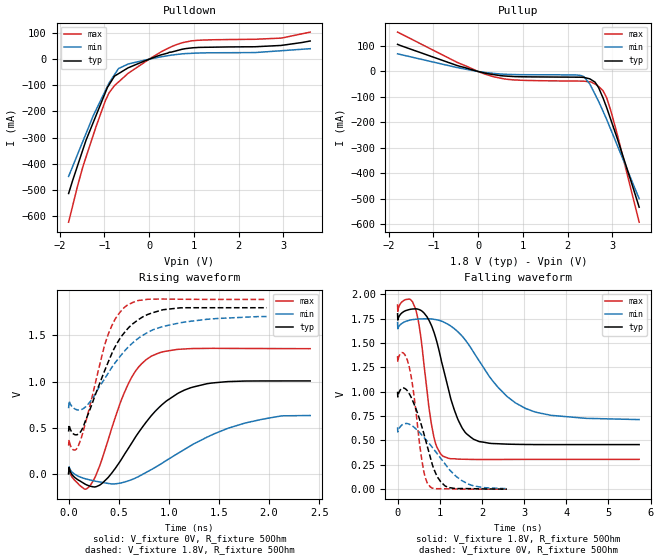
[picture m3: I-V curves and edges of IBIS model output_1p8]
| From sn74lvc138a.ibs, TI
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|   output_1p8 Model
[Model]   output_1p8
Model_type   Output
Polarity   Non-Inverting
Vmeas = 0.9
Vref = 0.9
Cref = 2pF
Rref = 50
|   typ   min   max
|   (nom PVT)   (fast PVT)   (slow PVT)
|C_comp from frequency sweep method (F=5MHz)
|C_comp   6.350e-12   6.256e-12   7.540e-12
|ON state : BUFFER OUTPUT TURNED HIGH
|C_comp   6.350e-12   6.256e-12   7.540e-12
|OFF state: BUFFER OUTPUT TURNED LOW
|C_comp   9.360e-12   9.345e-12   9.377e-12
|C_comp from LC tank measurement(L=1nH)
|Resonant Frequency(Hz)   2.130e+09   2.150e+09   2.080e+09
C_comp   5.589e-12   5.485e-12   5.861e-12
|ON state : BUFFER OUTPUT TURNED HIGH
|Resonant Frequency(Hz)   2.130e+09   2.150e+09   2.080e+09
|C_comp   5.589e-12   5.485e-12   5.861e-12
|OFF state: BUFFER OUTPUT TURNED LOW
|Resonant Frequency(Hz)   2.190e+09   2.210e+09   2.120e+09
|C_comp   5.287e-12   5.191e-12   5.642e-12
| Where nom  PVT is Nominal Process, 1.8V, 27C
|   Fast PVT is Strong Process,  1.89V, -40C
|   Slow PVT is Weak Process,   1.71V, 125C
[Voltage Range]   1.8   1.71   1.89
|Ambient Temperature   25   85   -40
|Junction Temperature
[Temperature Range]   27   125   -40
[Pullup Reference]   1.8   1.71   1.89
[Pulldown Reference]   0   0   0
[Power Clamp Reference]   1.8   1.71   1.89
[GND Clamp Reference]   0   0   0
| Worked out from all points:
|   slope of the pulldown table from 0 to 0.27 V, typ, clamps not added: 16.1 ohm
|   slope of the pullup table from 0 to 0.27 V, typ, clamps not added: 26.3 ohm
|   falling waveform, V_fixture 1.8V, R_fixture 50Ohm: 20-80 % time 503ps typ, 1.07ns min, 274ps max; typ from 1.8 V to 0.457 V
|   rising waveform, V_fixture 0V, R_fixture 50Ohm: 20-80 % time 446ps typ, 676ps min, 284ps max; typ from 0 V to 1.01 V
|   rising waveform, V_fixture 1.8V, R_fixture 50Ohm: 20-80 % time 335ps typ, 458ps min, 233ps max; typ from 0.457 V to 1.8 V
|   falling waveform, V_fixture 0V, R_fixture 50Ohm: 20-80 % time 412ps typ, 719ps min, 240ps max; typ from 1 V to 0 V
[Pulldown]
|   Voltage   I(typ)   I(min)   I(max)
-1.8V     -514.4mA   -448.9mA   -624.4mA
-1.482V   -347mA     -314.7mA   -412.2mA
-1.248V   -241.8mA   -216.2mA   -290.4mA
-980.9mV  -128.6mA   -121.3mA   -160mA
-897.8mV  -98.72mA   -91.84mA   -129.5mA
-774mV    -64.74mA   -59.18mA   -101.1mA
-685.7mV  -55.53mA   -36.01mA   -87.51mA
-470.6mV  -33.13mA   -18.62mA   -54.29mA
258.9mV   16.22mA    8.746mA    27.32mA
761.7mV   38.89mA    20.81mA    63.97mA
2.948V    52.67mA    32.41mA    80.78mA
3.6V      69.74mA    40.27mA    103.9mA
[Pullup]
|   Voltage   I(typ)   I(min)   I(max)
-1.8V     106.4mA    69.22mA    154.5mA
-470.6mV  23.41mA    15.43mA    35.98mA
332.6mV   -11.89mA   -7.173mA   -19.91mA
786.2mV   -19.78mA   -12.05mA   -32.97mA
2.291V    -22.48mA   -15.36mA   -37.74mA
2.367V    -23.31mA   -20.71mA   -37.9mA
2.497V    -28.83mA   -48.86mA   -40.43mA
2.663V    -55.08mA   -106.6mA   -54.04mA
2.79V     -102.6mA   -154.8mA   -74.48mA
2.871V    -140.4mA   -186.9mA   -102.1mA
2.967V    -189.6mA   -228.1mA   -154.2mA
3.6V      -532.3mA   -499.1mA   -591.2mA
[Ramp]
R_load = 50
|   typ   min   max
dV/dt_r   0.602271/4.41058e-10   0.391369/7.13501e-10   0.813764/2.83941e-10
dV/dt_f   0.805639/5.02765e-10   0.599447/1.06929e-09   0.950749/2.73761e-10
[Falling Waveform]
V_fixture = 1.8V
V_fixture_min = 1.71V
V_fixture_max = 1.89V
R_fixture = 50Ohm
|   Time   V(typ)   V(min)   V(max)
0s        1.8V       1.71V      1.89V
425ps     1.851V     1.744V     1.851V
540ps     1.838V     1.747V     1.599V
815ps     1.668V     1.746V     639.1mV
1.08ns    1.246V     1.718V     337.6mV
1.44ns    706.8mV    1.611V     307.9mV
1.935ns   488.3mV    1.316V     304.4mV
2.59ns    462mV      953.9mV    304.9mV
3.225ns   457.7mV    797.7mV    305.4mV
5.73ns    457.3mV    714.1mV    305.4mV
[Rising Waveform]
V_fixture = 0V
V_fixture_min = 0V
V_fixture_max = 0V
R_fixture = 50Ohm
|   Time   V(typ)   V(min)   V(max)
0s        108.6pV    12.82nV    54.42pV
5ps       69.56mV    74.84mV    62.58mV
115ps     -79.37mV   -35.53mV   -129.9mV
215ps     -134.8mV   -68.02mV   -127.7mV
390ps     -45.68mV   -104.4mV   351mV
590ps     265.1mV    -78.88mV   962.1mV
825ps     629.8mV    44.73mV    1.274V
1.09ns    871.4mV    220.5mV    1.349V
1.38ns    976.1mV    396.3mV    1.359V
2.41ns    1.006V     631.4mV    1.356V
[Rising Waveform]
V_fixture = 1.8V
V_fixture_min = 1.71V
V_fixture_max = 1.89V
R_fixture = 50Ohm
|   Time   V(typ)   V(min)   V(max)
0s        457.3mV    710.9mV    305.4mV
5ps       529.6mV    790.3mV    369.8mV
45ps      434.6mV    716.2mV    260.8mV
100ps     432.4mV    690.9mV    310.8mV
210ps     688.1mV    773.6mV    725.7mV
380ps     1.172V     1.065V     1.465V
465ps     1.379V     1.204V     1.677V
570ps     1.548V     1.345V     1.816V
945ps     1.779V     1.598V     1.894V
1.975ns   1.8V       1.704V     1.89V
[Falling Waveform]
V_fixture = 0V
V_fixture_min = 0V
V_fixture_max = 0V
R_fixture = 50Ohm
|   Time   V(typ)   V(min)   V(max)
0s        1V         634mV      1.366V
140ps     1.038V     668.7mV    1.397V
265ps     987.7mV    668.6mV    1.274V
370ps     895.4mV    642.6mV    1.022V
615ps     582.4mV    536.3mV    198.2mV
775ps     329.4mV    454.6mV    22.86mV
955ps     118.6mV    355.2mV    4.503mV
1.215ns   15.76mV    208mV      2.754mV
1.77ns    4.619mV    37.78mV    -323.4uV
2.595ns   108.5uV    4.387mV    -75.8uV
